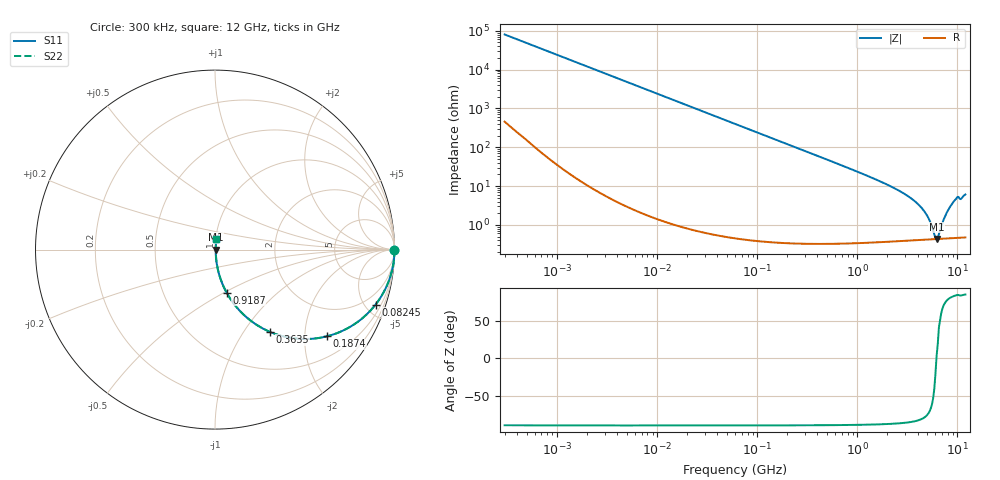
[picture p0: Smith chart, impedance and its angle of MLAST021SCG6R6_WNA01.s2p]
! MLAST021SCG6R6_WNA01  S-PARAMETER MODEL  ( General Type )
! Model Generated by TAIYO YUDEN Corporation (http://www.ty-top.com)
! Version 1.0
! TAIYO YUDEN Control No. 220901
! Copyright(c) 2022 TAIYO YUDEN CO.,LTD. All Rights Reserved.
! Product Description (link to TY-COMPAS)
! https://ds.yuden.co.jp/TYCOMPAS/or/detail?pn=MLAST021SCG6R6CWNA01&u=M
! Products Name : Multilayer Ceramic Capacitors
! Characteristics :
!  Capacitance : 6.6 pF , Rated Voltage : 25V , TCC : CG / C0G
!  Case Size : 0.25 x 0.125 / 0.0098 x 0.0049 [mm/inch] , Thickness : 0.125 / 0.0049 [mm/inch]
!  (Conditions: Temperature = 25 degC , DC Bias Current/Voltage = 0A / 0V)
! External Node Assignments :
!  1  o---| |---o  2
! GND o---------o GND
! Frequency Range : 0.3MHz  -  12000MHz  [ 401 STEP ]
# MHz S RI R 50
! Freq[MHz].  S11 Real  S11 Imag  S21 Real  S21 Imag  S12 Real  S12 Imag  S22 Real  S22 Imag
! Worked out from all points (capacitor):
!   401 points, 300 kHz to 12 GHz, reference 50 ohm
!   read as one part in series: C = 6.6 pF near 316.3 kHz
!   lowest |Z| = 433 mohm at 6.188 GHz (marker M1)
!   series resonance near 6.167 GHz, so ESL is about 100 pH
!   S11 on the Smith chart (normalised r, x): 300 kHz: open; 82.45 MHz: 1.01, -5.85; 187.4 MHz: 1.01, -2.57; 363.5 MHz: 1.01, -1.32; 918.7 MHz: 1.01, -0.51; 12 GHz: 1.01, +0.12
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0.3  1 -0.00124  8.6e-06 0.00124  8.6e-06 0.00124  1 -0.00124
1.769972  0.9999 -0.00734  6.07e-05 0.00734  6.07e-05 0.00734  0.9999 -0.00734
10.44266  0.9981 -0.0432  0.0019 0.0432  0.0019 0.0432  0.9981 -0.0432
27.10171  0.9874 -0.111  0.0126 0.111  0.0126 0.111  0.9874 -0.111
60  0.9415 -0.2342  0.0585 0.2342  0.0585 0.2342  0.9415 -0.2342
82.45425  0.895 -0.3059  0.105 0.3059  0.105 0.3059  0.895 -0.3059
187.4445  0.6226 -0.4834  0.3774 0.4834  0.3774 0.4834  0.6226 -0.4834
353.9943  0.3163 -0.4627  0.6837 0.4627  0.6837 0.4627  0.3163 -0.4627
363.4975  0.305 -0.458  0.695 0.458  0.695 0.458  0.305 -0.458
570.2811  0.1514 -0.3546  0.8486 0.3546  0.8486 0.3546  0.1514 -0.3546
918.7169  0.0645 -0.2393  0.9355 0.2393  0.9355 0.2393  0.0645 -0.2393
2088.533  0.0139 -0.1004  0.9861 0.1004  0.9861 0.1004  0.0139 -0.1004
3190.978  0.00691 -0.0547  0.9931 0.0547  0.9931 0.0547  0.00691 -0.0547
4270.516  0.00492 -0.029  0.9951 0.029  0.9951 0.029  0.00492 -0.029
5006.236  0.00444 -0.0162  0.9956 0.0162  0.9956 0.0162  0.00444 -0.0162
5868.704  0.00429 -0.00369  0.9957 0.00369  0.9957 0.00369  0.00429 -0.00369
6188.031  0.00431 0.000239  0.9957 -0.000239  0.9957 -0.000239  0.00431 0.000239
6524.734  0.00435 0.00379  0.9956 -0.00379  0.9956 -0.00379  0.00435 0.00379
7648.807  0.00475 0.0177  0.9952 -0.0177  0.9952 -0.0177  0.00475 0.0177
8732.115  0.00558 0.0325  0.9944 -0.0325  0.9944 -0.0325  0.00558 0.0325
9708.23  0.00675 0.0464  0.9933 -0.0464  0.9933 -0.0464  0.00675 0.0464
12000  0.00831 0.0597  0.9917 -0.0597  0.9917 -0.0597  0.00831 0.0597
